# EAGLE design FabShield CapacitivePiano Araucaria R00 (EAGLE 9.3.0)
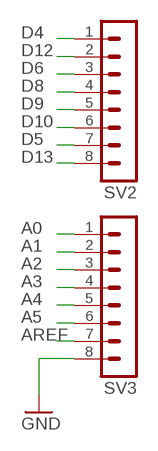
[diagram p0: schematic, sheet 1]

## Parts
SV2  MA08-1  [MA08-1]
SV3  MA08-1  [MA08-1]

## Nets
A0: SV3.1
A1: SV3.2
A2: SV3.3
A3: SV3.4
A4: SV3.5
A5: SV3.6
AREF: SV3.7
D4: SV2.1
D5: SV2.7
D6: SV2.3
D8: SV2.4
D9: SV2.5
D10: SV2.6
D12: SV2.2
D13: SV2.8
GND: SV3.8

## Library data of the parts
SV2 SV3 = con-lstb:MA08-1: PIN HEADER

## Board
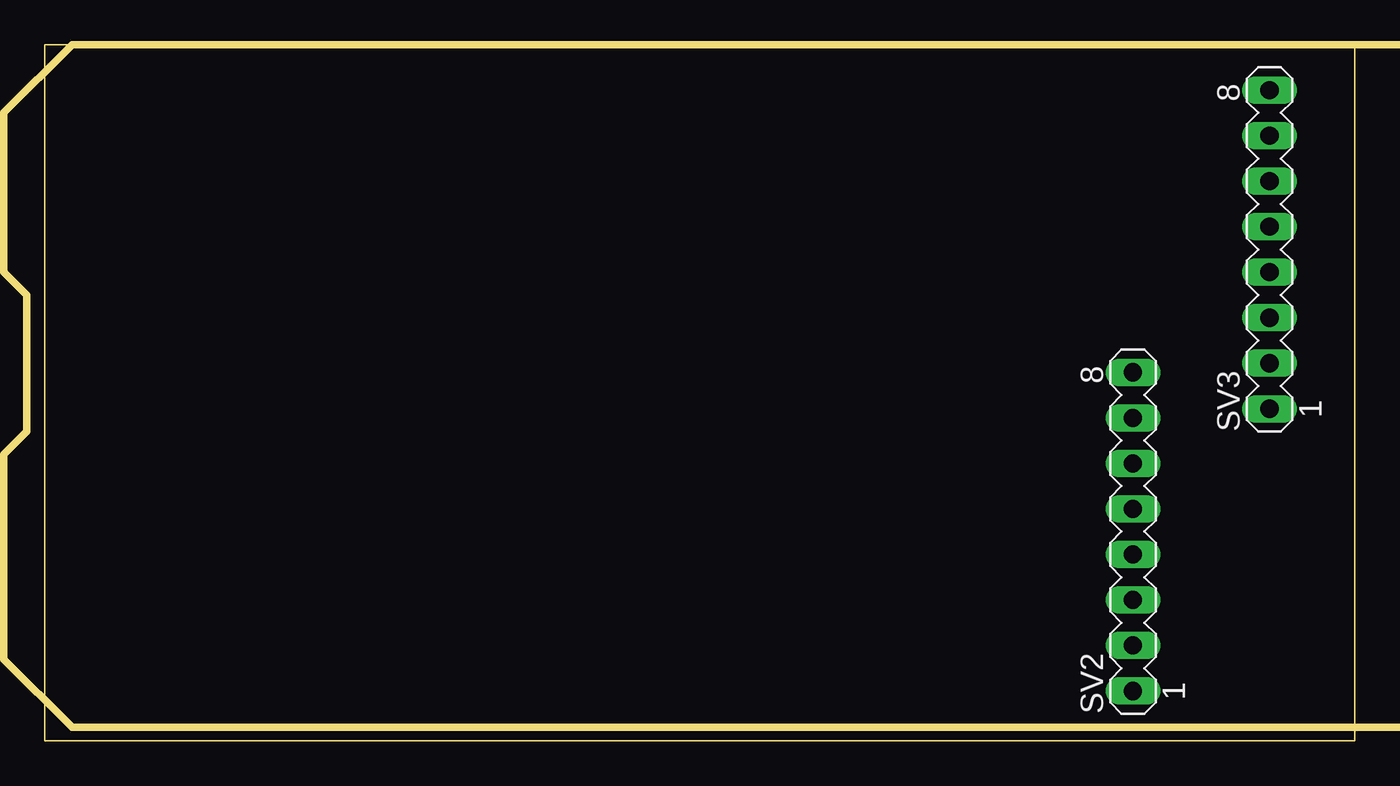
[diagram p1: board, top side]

Size 73.08 x 38.85 mm. Coordinates in mm from the lower left corner, seen from the top.
Outline: 0,0 73.08,0 73.08,38.85 0,38.85 0,0
Copper layers (1*16): Top 0.035mm / dielectric 1.5mm / Bottom 0.035mm
Design rules "default *": minimum track width 10mil, minimum drill 24mil, track to track 0.4mm, track to pad 0.4mm, pad to pad 0.4mm, via to via 0.4mm, smd to smd 0.4mm, copper to edge 40mil, drill to drill 0.4mm, minimum pad ring 10mil, minimum via ring 8mil, stop-mask expansion 4mil, vias tented up to drill 0mil, thermal gap 10mil
Milling: area -2.3,0.8 to 98,38.9

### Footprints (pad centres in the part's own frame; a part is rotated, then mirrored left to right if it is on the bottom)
MA08-1 = drill 1.016 long: 1 -8.89,0; 2 -6.35,0; 3 -3.81,0; 4 -1.27,0; 5 1.27,0; 6 3.81,0; 7 6.35,0; 8 8.89,0

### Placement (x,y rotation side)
SV2  60.71,11.68 90 top
SV3  68.33,27.43 90 top

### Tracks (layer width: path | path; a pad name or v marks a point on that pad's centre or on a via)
D13
  Top 0.305: SV2.8 60.96,20.57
